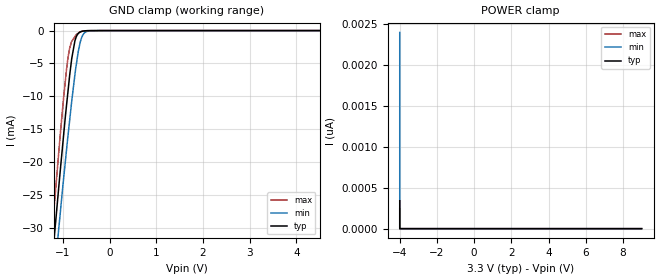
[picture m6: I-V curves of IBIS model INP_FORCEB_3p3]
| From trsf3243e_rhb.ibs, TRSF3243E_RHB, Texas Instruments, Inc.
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[Model]   INP_FORCEB_3p3
Model_type   Input
Vinl = 0.6
Vinh = 2.4
|   typ   min   max
C_comp   0.802pF	0.773pF	0.843pF
[Voltage Range]   3.3   3   3.6
[Temperature Range]   27   110   -40
[Power Clamp Reference]   3.3   3   3.6
[GND Clamp Reference]   0   0   0
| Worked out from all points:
|   GND clamp passes 1 mA (typ) near -0.72 V on its own axis
[GND Clamp]
|   Voltage   I(typ)   I(min)   I(max)
-4V       -268.4mA   -254.7mA   -282.4mA
-1.309V   -41.51mA   -46.48mA   -37.61mA
-1.186V   -31.55mA   -37.36mA   -26.74mA
-1.061V   -21.67mA   -28.11mA   -16.23mA
-889.4mV  -9.181mA   -15.93mA   -4.092mA
-809.3mV  -4.223mA   -10.68mA   -1.642mA
-742.4mV  -1.572mA   -6.738mA   -917.7uA
-672.8mV  -469.7uA   -3.285mA   -383.5uA
-598.7mV  -128.2uA   -1.088mA   -121.3uA
-491.9mV  -21.71uA   -138.5uA   -20.92uA
-230.8mV  -6.764uA   -244.3nA   -2.254uA
9V        0A         0A         0A
[POWER Clamp]
|   Voltage   I(typ)   I(min)   I(max)
-4V       340.5pA    2.399nA    246.8pA
-4V       0A         0A         0A
-4V       0A         0A         0A
9V        0A         0A         0A
